TYPE ST_MemoryData :
STRUCT
	(* Single points *)
	eSPI_100_msg		: E_IEC870_5_101SPI;
	eSPI_101_msg		: E_IEC870_5_101SPI;
	eSPI_102_msg		: E_IEC870_5_101SPI;

	(* Double points *)
	eDPI_200_msg		: E_IEC870_5_101DPI;
	eDPI_201_msg		: E_IEC870_5_101DPI;
	eDPI_202_msg		: E_IEC870_5_101DPI;

	(* Regulating step values *)
	nVTI_300_msg		: BYTE;
	nVTI_301_msg		: BYTE;
	nVTI_302_msg		: BYTE;

	(* 32 bit strings *)
	nBSI_400_msg 		: DWORD;
	nBSI_401_msg 		: DWORD;
	nBSI_402_msg		: DWORD;

	(* Measured values, normalized values *)
	nNVA_500_msg		: WORD;
	nNVA_501_msg		: WORD;
	nNVA_502_msg		: WORD;

	(* Mesured values, scaled values *)
	nSVA_600_msg		: INT;
	nSVA_601_msg		: INT;
	nSVA_602_msg		: INT;

	(* Measured values, short floating point values *)
	fR32_700_msg		: REAL;
	fR32_701_msg		: REAL;
	fR32_702_msg		: REAL;

	(* Integrated totals *)
	nBCR_800_msg		: UDINT;
	nBCR_801_msg		: UDINT;
	nBCR_802_msg		: UDINT;

	(*#################################################################*)
	(* Single commands *)
	eSCS_10_cmd			: E_IEC870_5_101SCS;
	eSCS_11_cmd			: E_IEC870_5_101SCS;
	eSCS_12_cmd			: E_IEC870_5_101SCS;

	(* Double commands *)
	eDCS_20_cmd			: E_IEC870_5_101DCS;
	eDCS_21_cmd			: E_IEC870_5_101DCS;
	eDCS_22_cmd			: E_IEC870_5_101DCS;

	(* Regulating step commands *)
	eRCS_30_cmd			: E_IEC870_5_101RCS;
	eRCS_31_cmd			: E_IEC870_5_101RCS;
	eRCS_32_cmd			: E_IEC870_5_101RCS;
	
	(* 32 bit string commands *)
	nBSI_40_cmd			: DWORD;
	nBSI_41_cmd			: DWORD;
	nBSI_42_cmd			: DWORD;

	(* Set point, normalized values *)
	nNVA_50_cmd			: WORD;
	nNVA_51_cmd			: WORD;
	nNVA_52_cmd			: WORD;

	(* Set point, scaled values *)
	nSVA_60_cmd			: INT;
	nSVA_61_cmd			: INT;
	nSVA_62_cmd			: INT;

	(* Set point, short floating point values *)
	fR32_70_cmd			: REAL;
	fR32_71_cmd			: REAL;
	fR32_72_cmd			: REAL;
	
END_STRUCT
END_TYPE
